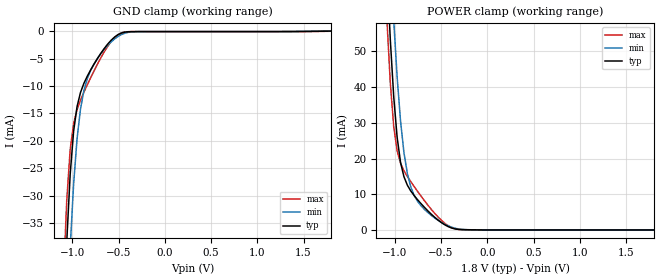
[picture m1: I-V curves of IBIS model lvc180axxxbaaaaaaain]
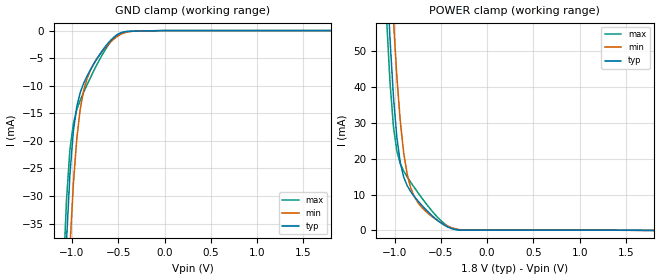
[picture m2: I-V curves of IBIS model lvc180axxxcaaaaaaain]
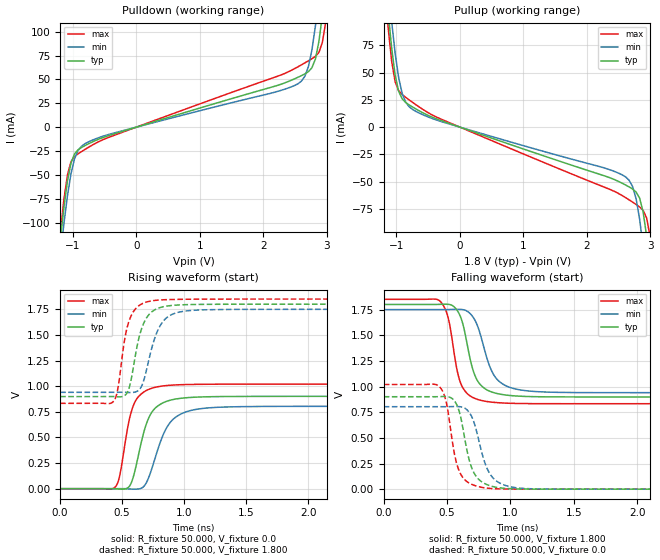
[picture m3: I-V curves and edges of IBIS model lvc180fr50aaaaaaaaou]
| IBIS Models Generator: Lattice Radiant Software (64-bit) 2023.2.t.305.0
| Report Generate Date: Mar 14 2024
| Report Generate Time: 15:47:07
| IBIS File LibisMaker.ibs
| Cadence Design Systems, Inc. 2022
[IBIS Ver]   7.1
[File Name]   Blink_RevB_impl_1.ibs
[File rev]   0.8
[Date]   Wed Oct 26 21:07:21 PDT 2022
[Source]   Lattice Semiconductor Process
   Lattice Semiconductor has worked hard to ensure the
   models below are accurate and complete.  However, the
   data below was generated using simulation of the
   input/output model files for the silicon.  Therefore,
   the data below is for reference and initial design
   purposes only.
   Lattice Semiconductor grants permission to use this
   data for use in printed circuit design using this
   Lattice programmable logic device.  Other use of this
   code, including the selling or duplication of any
   portion is strictly prohibited.
|   NAMING CONVENTION
   The IBIS [Model] header is limited by the specification to a
   total of characters.  With such a set of characters available
   for naming models it becomes important to attempt to
   meaningfully encode the IO standards so they fit within the
   twenty character limit.  It would seem that twenty characters
   would provide room enough for describing IO's.  However, the
   PLD IO structure continues to grow more and more complex.  The
   complexity is making the twenty characters insuffiently
   descriptive.  In order to overcome this issue the naming
   convention described below is implemented to resolve the issue.
The twenty character space is managed as follows:
   bbbvvvsdddprttakoixx
   b = standard
   v = voltage (x.xx V)
   s = slew code
   d = drive (xx.x ma)
   p = pullmode code
   r = impedance
   t = termination code
   k = bank code
   o = diff resistor code
   i = diff  current code
   x = reserved
   standard
   lvcmos   lvc
   sstl135   ss1
   sstl135d   s1d
   hsul12   hs1
   hsul12d   h1d
   lvds   lvs
   lvdse   lve
   slvs   svs
   sublvds   slv
   sublvdse   sle
   mipi_dphy   mip
   pod   pod
   podd   pdd
   lvstl_i   ls1
   lvstl_ii   ls2
   lvstld_i   l1d
   lvstld_ii   l2d
   vref_driver   vr1
   slew
   na   a
   fast   f
   slow   s
   drive
   2   020
   4   040
   6   060
   8   080
   12   120
   50rs   r50
   34_ohm   034
   40_ohm   040
   48_ohm   048
   60_ohm   060
   80_ohm   080
   120_ohm   120
   240_ohm   240
   na   xxx
   pullmode
   none   a
   failsafe   a
   up   b
   down   c
   keeper   d
   i3c   i
   impedance
   off   a
   termination
   off   aa
   34   bb
   40   cc
   48   dd
   60   ee
   80   ff
   120   gg
   240   hh
   bank
   wrio   a
   hpio   h
   differential resistor
   off   a
   100   b
   differential current
   NA   a
   2   b
   3.5   c
   Reserved   IO type
   in   input only
   ou   output
   io   I/O
   od   Open drain
   on   Inverting differential I/O
   (signal name only)
   op   Non-Inverting differential I/O
   (signal name only)
   All the IO models are generated with pull mode set to none.
   Lattice Semiconductor Corporation
   5555 NE Moore Court
   Hillsboro, OR 97214
   U.S.A
   TEL: 1-800-Lattice (USA and Canada)
   408-826-6000 (other locations)
   web: http://www.latticesemi.com/
   email: techsupport@latticesemi.com
[Disclaimer] This IBIS source code is intended as a design reference
   which illustrates how the Lattice Semiconductor device operates.
   It is the user's responsibility to verify their design for
   consistency and functionality through the use of formal
   verification methods.  Lattice Semiconductor provides no warranty
   regarding the use or functionality of this data.
[Copyright]   Copyright 2022 by Lattice Semiconductor Corporation
|   Component LAV-AT
[Component] LAV-AT
[Manufacturer] Lattice Semiconductor Corp.
[Package]
|LFG1156
| variable   typ   min   max
R_pkg   0.71222   0.080273   1.4611
L_pkg   4.484e-9   6.708e-10   8.258e-9
C_pkg   2.172e-12   8.235e-13   3.735e-12
[Pin]  signal_name   model_name   R_pin   L_pin   C_pin
T7   clk_in   lvc330axxxcaaaaaaain
V16   sw12   lvc330axxxcaaaaaaain
V15   sw13   lvc330axxxcaaaaaaain
T13   sw14   lvc330axxxcaaaaaaain
R13   sw15   lvc330axxxcaaaaaaain
R19   seg1   lvc330sr50aaaaaaaaou
R18   seg2   lvc330sr50aaaaaaaaou
R14   seg3   lvc330sr50aaaaaaaaou
T18   seg_a   lvc330sr50aaaaaaaaou
T19   seg_b   lvc330sr50aaaaaaaaou
T15   seg_c   lvc330sr50aaaaaaaaou
U16   seg_d   lvc330sr50aaaaaaaaou
U17   seg_e   lvc330sr50aaaaaaaaou
W14   seg_f   lvc330sr50aaaaaaaaou
V14   seg_g   lvc330sr50aaaaaaaaou
R15   seg_dp   lvc330sr50aaaaaaaaou
L11   MDQ1   lvc180fr50baaaaaaaio
P2   PROGRAMN   lvc180axxxbaaaaaaain
L12   MDQ0   lvc180fr50baaaaaaaio
P1   CFGMODE   lvc180axxxbaaaaaaain
R1   TMS   lvc180axxxbaaaaaaain
R7   ERASEKEY   lvc180axxxcaaaaaaain
P9   MCLKP   lvc180fr50aaaaaaaaou
T5   INITN   lvc180fr50baaaaaaaio
U1   TDI   lvc180axxxbaaaaaaain
P7   MCSN   lvc180fr50aaaaaaaaou
T1   TCK   lvc180axxxcaaaaaaain
U5   SSDO   lvc180fr50aaaaaaaaou
U4   DONE   lvc180fr50baaaaaaaio
U2   TDO   lvc180fr50aaaaaaaaou
| Models and submodels in the file (5): lvc180axxxbaaaaaaain (Input), lvc180axxxcaaaaaaain (Input), lvc180fr50aaaaaaaaou (Output), lvc330axxxcaaaaaaain (Input), lvc330sr50aaaaaaaaou (Output)
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[Model] lvc180axxxbaaaaaaain
Model_type Input
Polarity   Non-Inverting
Enable   Active-High
Vinl =  0.630V
Vinh =  1.170V
C_comp   5.000pF   4.000pF   5.500pF
[Temperature Range]   25.000   0.125k   -40.000
[Voltage Range]   1.800V   1.710V   1.890V
[C Comp Corner]
C_comp   5.000pF   4.000pF   5.500pF
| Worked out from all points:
|   GND clamp passes 1 mA (typ) near -0.54 V on its own axis
|   POWER clamp passes 1 mA (typ) near -0.43 V on its own axis
[GND_clamp]
|Voltage   I(typ)   I(min)   I(max)
-1.8V     -585.7mA   -591.6mA   -585.2mA
-1.097V   -54.7mA    -72.3mA    -45.45mA
-1.06V    -38.25mA   -54.4mA    -30.74mA
-1.023V   -26.05mA   -39.45mA   -21.57mA
-986mV    -18.23mA   -27.85mA   -16.83mA
-949mV    -13.77mA   -19.64mA   -14.31mA
-912mV    -11.21mA   -14.25mA   -12.59mA
-875mV    -9.522mA   -10.85mA   -11.14mA
-727mV    -4.965mA   -4.951mA   -5.982mA
-505mV    -637.4uA   -970.5uA   -652uA
-320mV    -95.22uA   -117uA     -94.3uA
1.8V      -11.32nA   0A         -27.08uA
[POWER_clamp]
|Voltage   I(typ)   I(min)   I(max)
-1.789V   650.9mA    666.7mA    643.9mA
-1.086V   73.39mA    99.35mA    59.12mA
-1.049V   53.39mA    77.75mA    41.23mA
-1.012V   37.33mA    58.72mA    28.99mA
-975mV    25.93mA    42.82mA    22.15mA
-938mV    18.88mA    30.44mA    18.65mA
-901mV    14.88mA    21.58mA    16.56mA
-827mV    10.9mA     12.02mA    13.52mA
-716mV    7.349mA    6.758mA    9.453mA
-457mV    1.407mA    1.574mA    1.826mA
-272mV    92.84uA    154.7uA    100.2uA
1.8V      0A         0A         0A
[Model] lvc180axxxcaaaaaaain
Model_type Input
Polarity   Non-Inverting
Enable   Active-High
Vinl =  0.630V
Vinh =  1.170V
C_comp   5.000pF   4.000pF   5.500pF
[Temperature Range]   25.000   0.125k   -40.000
[Voltage Range]   1.800V   1.710V   1.890V
[C Comp Corner]
C_comp   5.000pF   4.000pF   5.500pF
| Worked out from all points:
|   GND clamp passes 1 mA (typ) near -0.53 V on its own axis
|   POWER clamp passes 1 mA (typ) near -0.43 V on its own axis
[GND_clamp]
|Voltage   I(typ)   I(min)   I(max)
-1.8V     -585.7mA   -591.6mA   -585.2mA
-1.097V   -54.72mA   -72.31mA   -45.48mA
-1.06V    -38.27mA   -54.42mA   -30.77mA
-1.023V   -26.08mA   -39.46mA   -21.61mA
-986mV    -18.26mA   -27.87mA   -16.88mA
-949mV    -13.8mA    -19.66mA   -14.36mA
-912mV    -11.24mA   -14.28mA   -12.64mA
-875mV    -9.559mA   -10.88mA   -11.19mA
-727mV    -5.003mA   -4.978mA   -6.034mA
-505mV    -676uA     -991uA     -711.7uA
-283mV    -81.53uA   -79.99uA   -96.61uA
1.8V      0A         0A         0A
[POWER_clamp]
|Voltage   I(typ)   I(min)   I(max)
-1.789V   650.9mA    666.7mA    643.9mA
-1.086V   73.38mA    99.34mA    59.1mA
-1.049V   53.37mA    77.74mA    41.21mA
-1.012V   37.32mA    58.71mA    28.96mA
-975mV    25.91mA    42.81mA    22.12mA
-938mV    18.86mA    30.42mA    18.62mA
-901mV    14.86mA    21.57mA    16.53mA
-827mV    10.88mA    12mA       13.48mA
-716mV    7.324mA    6.743mA    9.419mA
-457mV    1.39mA     1.57mA     1.798mA
-272mV    110.1uA    181.6uA    103uA
1.8V      0A         0A         27.97uA
[Model] lvc180fr50aaaaaaaaou
Model_type Output
Polarity   Non-Inverting
Enable   Active-High
Vmeas =  0.900V
Cref =  0.0F
Rref =  1.000M
Vref =  0.0V
C_comp   2.000pF   1.500pF   2.500pF
[Temperature Range]   25.000   0.125k   -40.000
[Voltage Range]   1.800V   1.750V   1.850V
[C Comp Corner]
C_comp   2.000pF   1.500pF   2.500pF
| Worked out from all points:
|   slope of the pulldown table from 0 to 0.27 V, typ, clamps not added: 49.6 ohm
|   slope of the pullup table from 0 to 0.27 V, typ, clamps not added: 49.6 ohm
|   rising waveform, R_fixture 50.000, V_fixture 0.0: 20-80 % time 123ps typ, 156ps min, 99.8ps max; typ from 0 V to 0.901 V
|   rising waveform, R_fixture 50.000, V_fixture 1.800: 20-80 % time 101ps typ, 121ps min, 85.3ps max; typ from 0.899 V to 1.8 V
|   falling waveform, R_fixture 50.000, V_fixture 1.800: 20-80 % time 108ps typ, 133ps min, 93.2ps max; typ from 1.8 V to 0.899 V
|   falling waveform, R_fixture 50.000, V_fixture 0.0: 20-80 % time 100ps typ, 118ps min, 88.7ps max; typ from 0.901 V to 0 V
[Pulldown]
|Voltage   I(typ)   I(min)   I(max)
-1.8V     -588.1mA   -593.7mA   -587.9mA
-1.195V   -117.3mA   -134mA     -108.8mA
-1.14V    -83.87mA   -100.8mA   -75.47mA
-1.085V   -56.41mA   -71.92mA   -50.09mA
-975mV    -28.18mA   -33.55mA   -30.9mA
-810mV    -19.37mA   -17.42mA   -23.41mA
2.49V     50.62mA    43.58mA    61.28mA
2.71V     58.22mA    63.6mA     69.54mA
2.82V     71.46mA    106.2mA    74.21mA
2.93V     118.1mA    173.4mA    89.03mA
2.985V    153mA      212.4mA    111.8mA
3.6V      665.6mA    724.8mA    614.6mA
[Pullup]
|Voltage   I(typ)   I(min)   I(max)
-1.8V     662mA      677.7mA    655.3mA
-1.13V    105.1mA    130.9mA    90.99mA
-1.075V   72.43mA    96.72mA    60.56mA
-1.02V    47.64mA    67.65mA    41.57mA
-910mV    25.97mA    30.95mA    29.89mA
-745mV    18.4mA     16.18mA    22.67mA
2.5V      -49.81mA   -42.2mA    -60.87mA
2.72V     -56.75mA   -54.52mA   -68.72mA
2.885V    -77.69mA   -109.9mA   -76.19mA
2.94V     -99.91mA   -140.9mA   -83.15mA
2.995V    -129.9mA   -175.4mA   -100.3mA
3.6V      -593.7mA   -639mA     -553.1mA
[Ramp]
| variable   typ   min   max
dV/dt_r   0.541/0.123n   0.482/0.156n   0.612/99.787p
dV/dt_f   0.541/0.108n   0.486/0.133n   0.610/93.264p
R_load = 50.000
[Rising Waveform]
R_fixture= 50.000
V_fixture= 0.0
V_fixture_min= 0.0
V_fixture_max= 0.0
|time   V(typ)   V(min)   V(max)
0s        360.1nV    3.438uV    103nV
448ps     -926.3uV   -9.701uV   21.92mV
485ps     -4.496mV   90.87uV    156mV
569ps     45.28mV    -3.423mV   730.8mV
607ps     195.8mV    -4.494mV   855.4mV
659ps     478mV      7.454mV    929.5mV
741ps     749.3mV    203.3mV    980.7mV
867ps     855.9mV    611.8mV    1.007V
1.075ns   891.9mV    769mV      1.017V
50ns      900.9mV    803.6mV    1.02V
[Rising Waveform]
R_fixture= 50.000
V_fixture= 1.800
V_fixture_min= 1.750
V_fixture_max= 1.850
|time   V(typ)   V(min)   V(max)
0s        898.6mV    940.1mV    832.7mV
433ps     898.7mV    940.3mV    856.2mV
464ps     896.2mV    940.4mV    967.7mV
515ps     905.5mV    940.4mV    1.419V
549ps     957.5mV    938.6mV    1.612V
630ps     1.445V     957.8mV    1.781V
697ps     1.668V     1.164V     1.821V
795ps     1.763V     1.565V     1.84V
955ps     1.792V     1.722V     1.847V
50ns      1.8V       1.75V      1.85V
[Falling Waveform]
R_fixture= 50.000
V_fixture= 1.800
V_fixture_min= 1.750
V_fixture_max= 1.850
|time   V(typ)   V(min)   V(max)
0s        1.8V       1.75V      1.85V
446ps     1.801V     1.75V      1.83V
511ps     1.801V     1.75V      1.657V
582ps     1.737V     1.752V     1.141V
657ps     1.421V     1.735V     933.5mV
704ps     1.163V     1.678V     892.8mV
765ps     1.015V     1.496V     866.1mV
874ps     938.5mV    1.102V     845.4mV
1.052ns   907.4mV    973mV      835.2mV
50ns      898.5mV    940.1mV    832.7mV
[Falling Waveform]
R_fixture= 50.000
V_fixture= 0.0
V_fixture_min= 0.0
V_fixture_max= 0.0
|time   V(typ)   V(min)   V(max)
0s        900.9mV    803.6mV    1.02V
446ps     902.1mV    803.6mV    990.4mV
495ps     902.5mV    803.6mV    837.7mV
568ps     841.8mV    805.6mV    287.2mV
643ps     466.3mV    786.6mV    87.72mV
685ps     240.4mV    727.7mV    52.26mV
735ps     115.3mV    551.8mV    29mV
825ps     39.23mV    177.1mV    9.064mV
955ps     8.109mV    38.24mV    1.629mV
50ns      3.598uV    9.764uV    1.615uV
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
